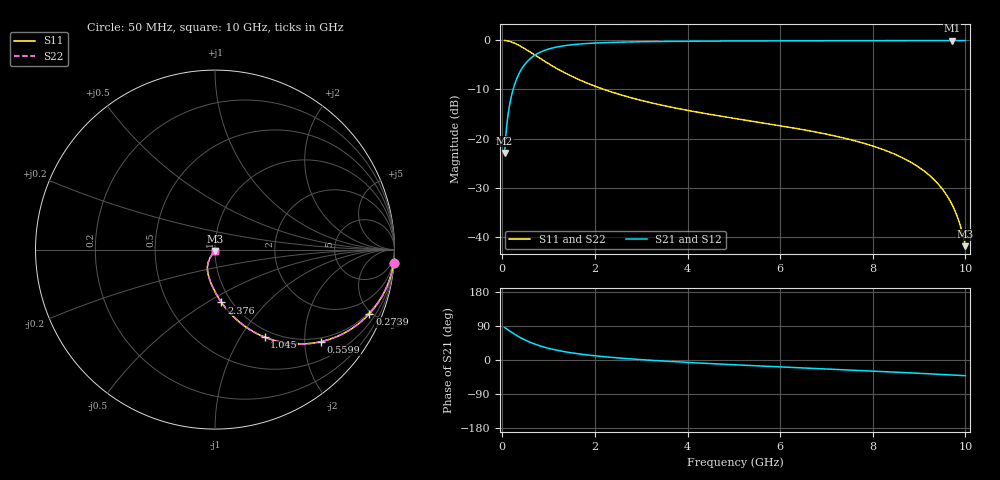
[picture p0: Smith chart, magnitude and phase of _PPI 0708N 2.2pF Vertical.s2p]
! S-Parameter data specifications (vertical orientation):
! Substrate: 40-mil Rogers 3003C, Substrate thickness, H=1.016mm, Dielectric constant, Er=3, Conductor thickness, T_mtl=0.043mm, Loss Tangent, Tand=0.003
! PCB Mounting Pad Footprint: Pad width, PadW=2.54mm , Pad length, PadL=0.51mm , Pad gap, PadG (edge-to-edge)=0.71mm , Reference planes=1.73mm apart
! Created Tue Jan 16 08:44:28 2018
# GHz S MA R 50
! 2 Port Network Data from SP1.SP block
! freq  magS11  angS11  magS21  angS21  magS12  angS12  magS22  angS22
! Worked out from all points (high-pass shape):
!   801 points, 50 MHz to 10 GHz, reference 50 ohm
!   highest |S21| = -0.04 dB at 9.714 GHz (marker M1); lowest = -22.9 dB at 50 MHz (marker M2)
!   |S21| within 3 dB of the highest: 699.1 MHz to end of sweep
!   lowest |S11| = -41.9 dB at 10 GHz (marker M3), VSWR 1.02, Z = 49.9 - j0.79 ohm
!   |S11| at or under -10 dB: 2.197 GHz to end of sweep
!   |S22| runs from -41.9 to 0.0 dB; largest |S21 - S12| = 0
!   S11 on the Smith chart (normalised r, x): 50 MHz: 1, -27; 273.9 MHz: 0.90, -4.85; 559.9 MHz: 0.90, -2.38; 1.045 GHz: 0.90, -1.28; 2.376 GHz: 0.90, -0.58; 10 GHz: 1.00, -0.02
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0.05  0.9975 -4.3  0.07128 85.7  0.07128 85.7  0.9975 -4.3
0.124625  0.9845 -10.6  0.1753 79.3  0.1753 79.3  0.9845 -10.6
0.1619375  0.9742 -13.7  0.2254 76.2  0.2254 76.2  0.9742 -13.7
0.273875  0.9312 -22.6  0.3642 67.4  0.3642 67.4  0.9312 -22.6
0.39825  0.8693 -31.4  0.494 58.6  0.494 58.6  0.8693 -31.4
0.5599375  0.7816 -41.0  0.6234 48.9  0.6234 48.9  0.7816 -41.0
0.79625  0.6623 -52.0  0.7487 38.0  0.7487 38.0  0.6623 -52.0
1.045  0.5604 -60.5  0.8275 29.5  0.8275 29.5  0.5604 -60.5
1.3435  0.4683 -67.9  0.8827 22.0  0.8827 22.0  0.4683 -67.9
1.716625  0.3868 -74.7  0.9212 15.2  0.9212 15.2  0.3868 -74.7
2.375812  0.2964 -83.0  0.9538 6.8  0.9538 6.8  0.2964 -83.0
3.370812  0.2224 -91.6  0.9734 -1.9  0.9734 -1.9  0.2224 -91.6
5.025  0.1601 -102.0  0.9851 -12.7  0.9851 -12.7  0.1601 -102.0
6.691625  0.1184 -110.9  0.9904 -22.0  0.9904 -22.0  0.1184 -110.9
7.624437  0.09456 -115.5  0.9925 -27.2  0.9925 -27.2  0.09456 -115.5
8.345812  0.07341 -118.9  0.9939 -31.2  0.9939 -31.2  0.07341 -118.9
8.818437  0.05751 -120.7  0.9947 -34.0  0.9947 -34.0  0.05751 -120.7
9.191562  0.04347 -121.5  0.9951 -36.3  0.9951 -36.3  0.04347 -121.5
9.490063  0.03112 -121.0  0.9953 -38.1  0.9953 -38.1  0.03112 -121.0
9.713938  0.02117 -118.6  0.9954 -39.5  0.9954 -39.5  0.02117 -118.6
9.85075  0.01483 -114.1  0.9953 -40.4  0.9953 -40.4  0.01483 -114.1
10  0.008016 -98.8  0.9953 -41.4  0.9953 -41.4  0.008016 -98.8
